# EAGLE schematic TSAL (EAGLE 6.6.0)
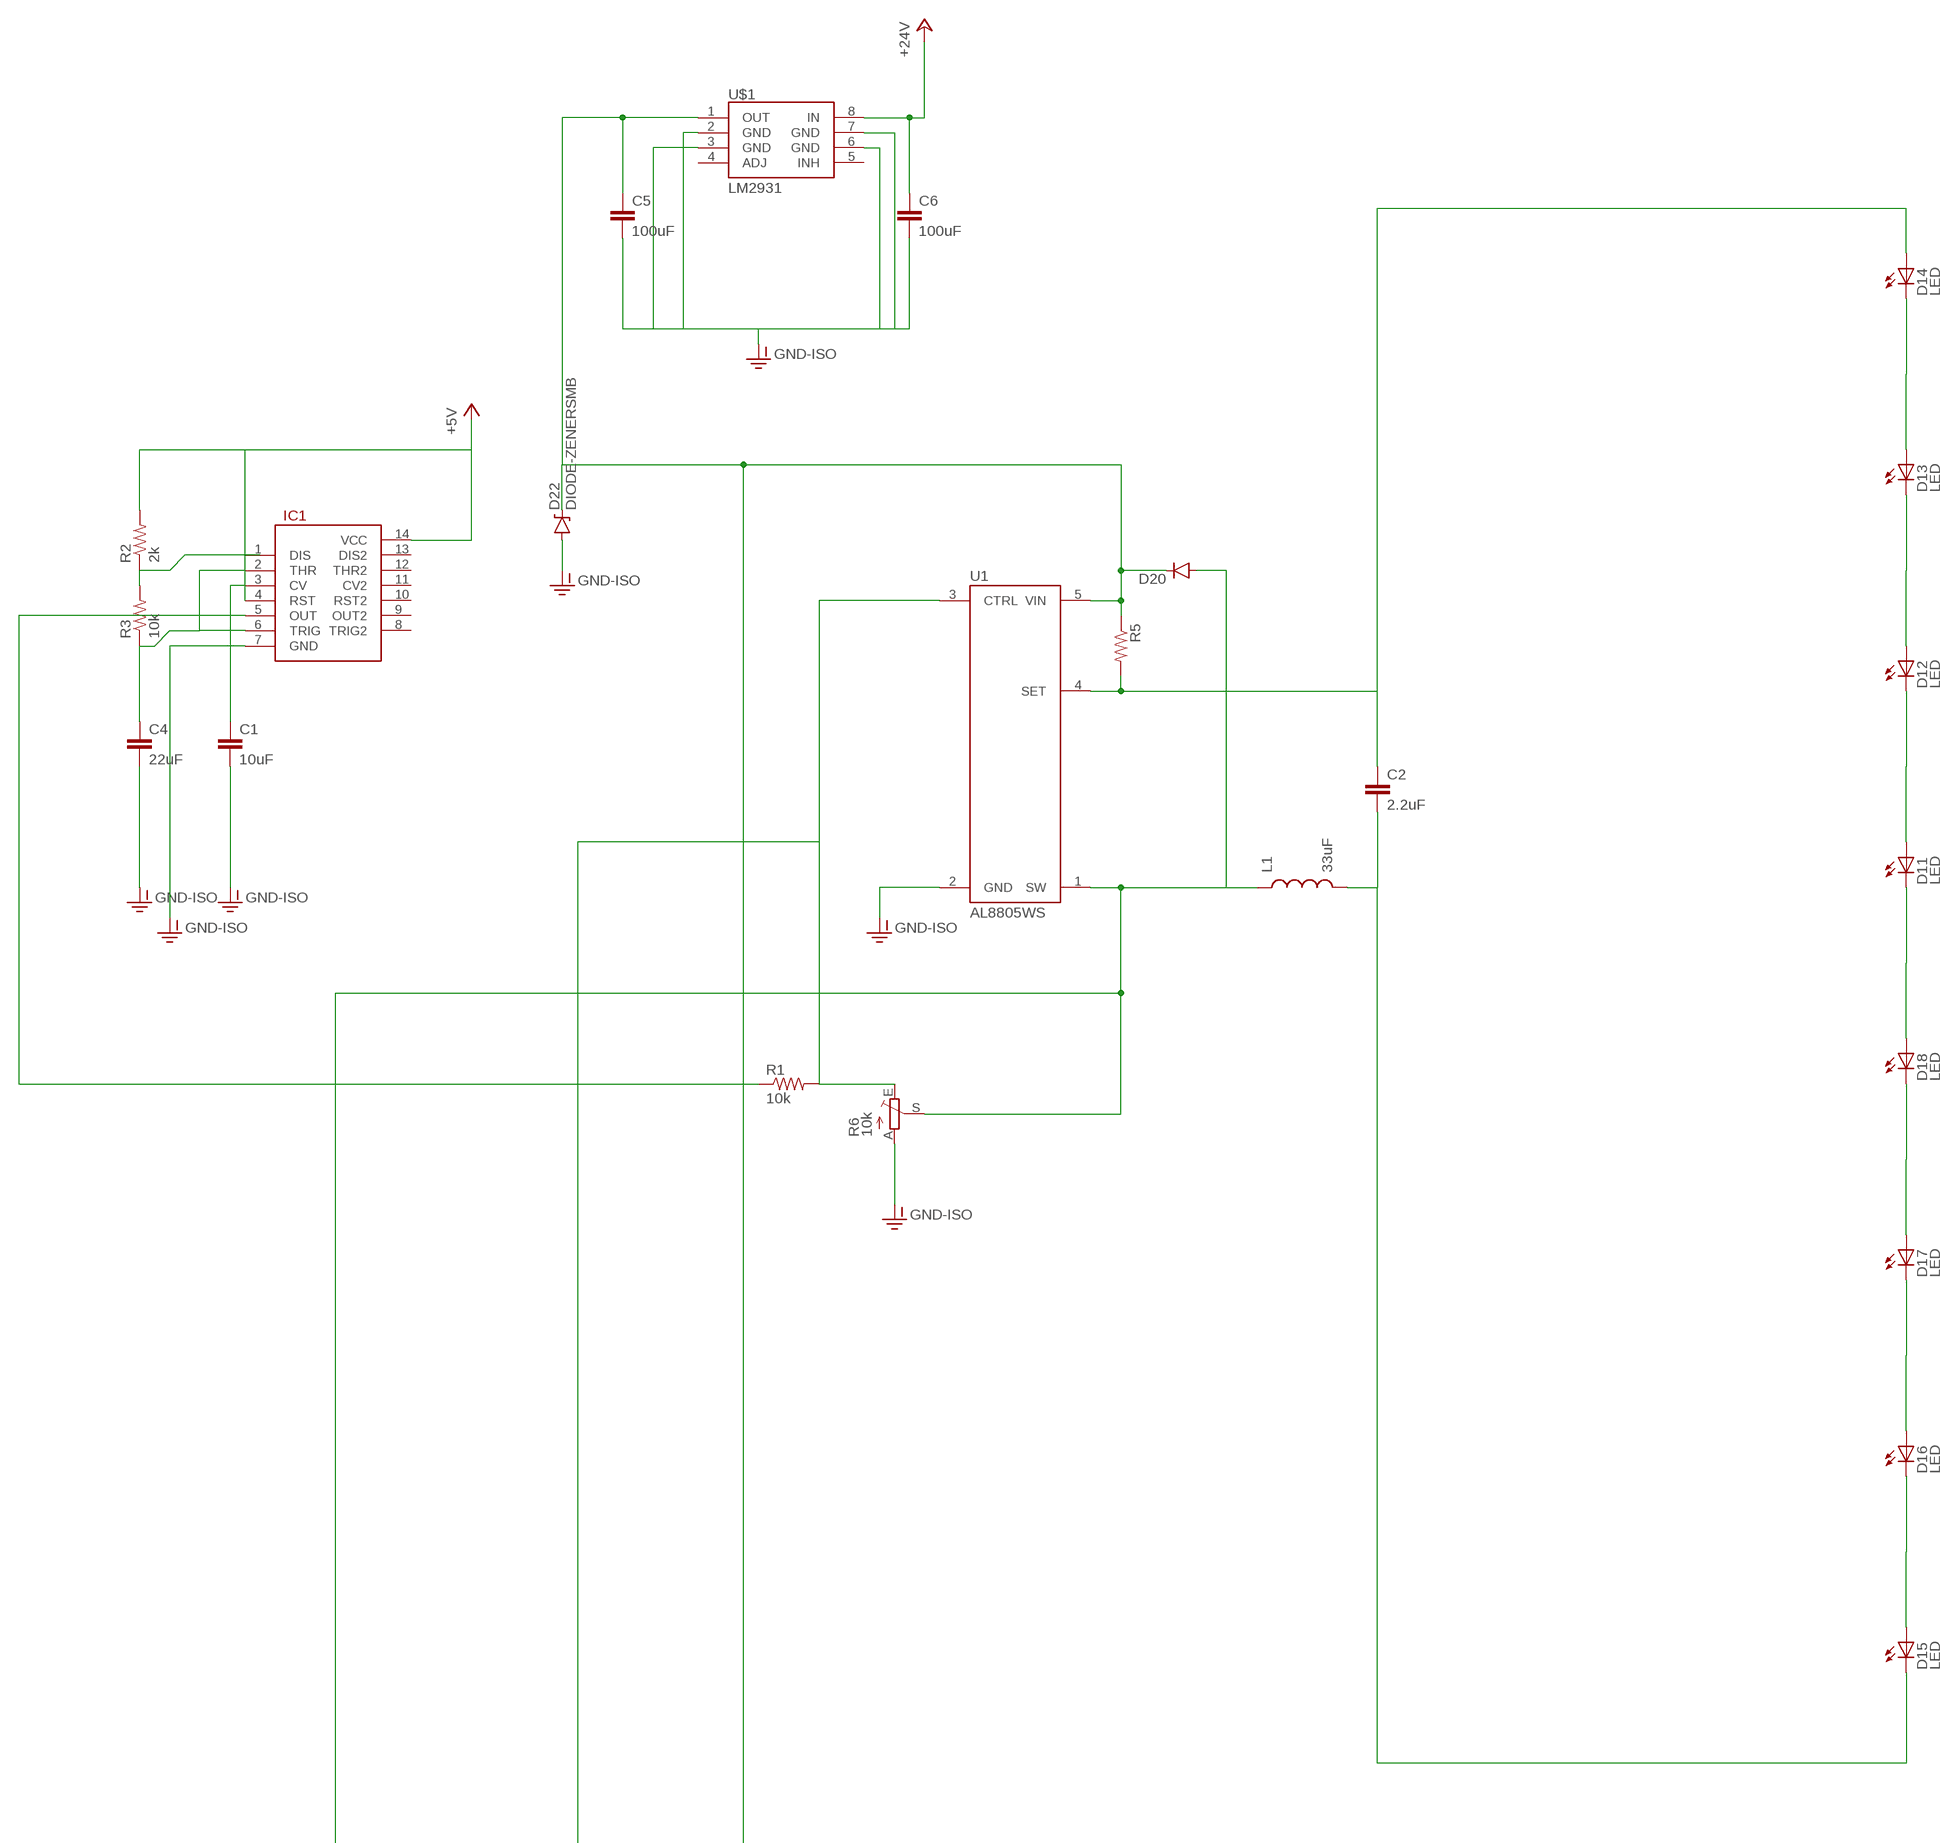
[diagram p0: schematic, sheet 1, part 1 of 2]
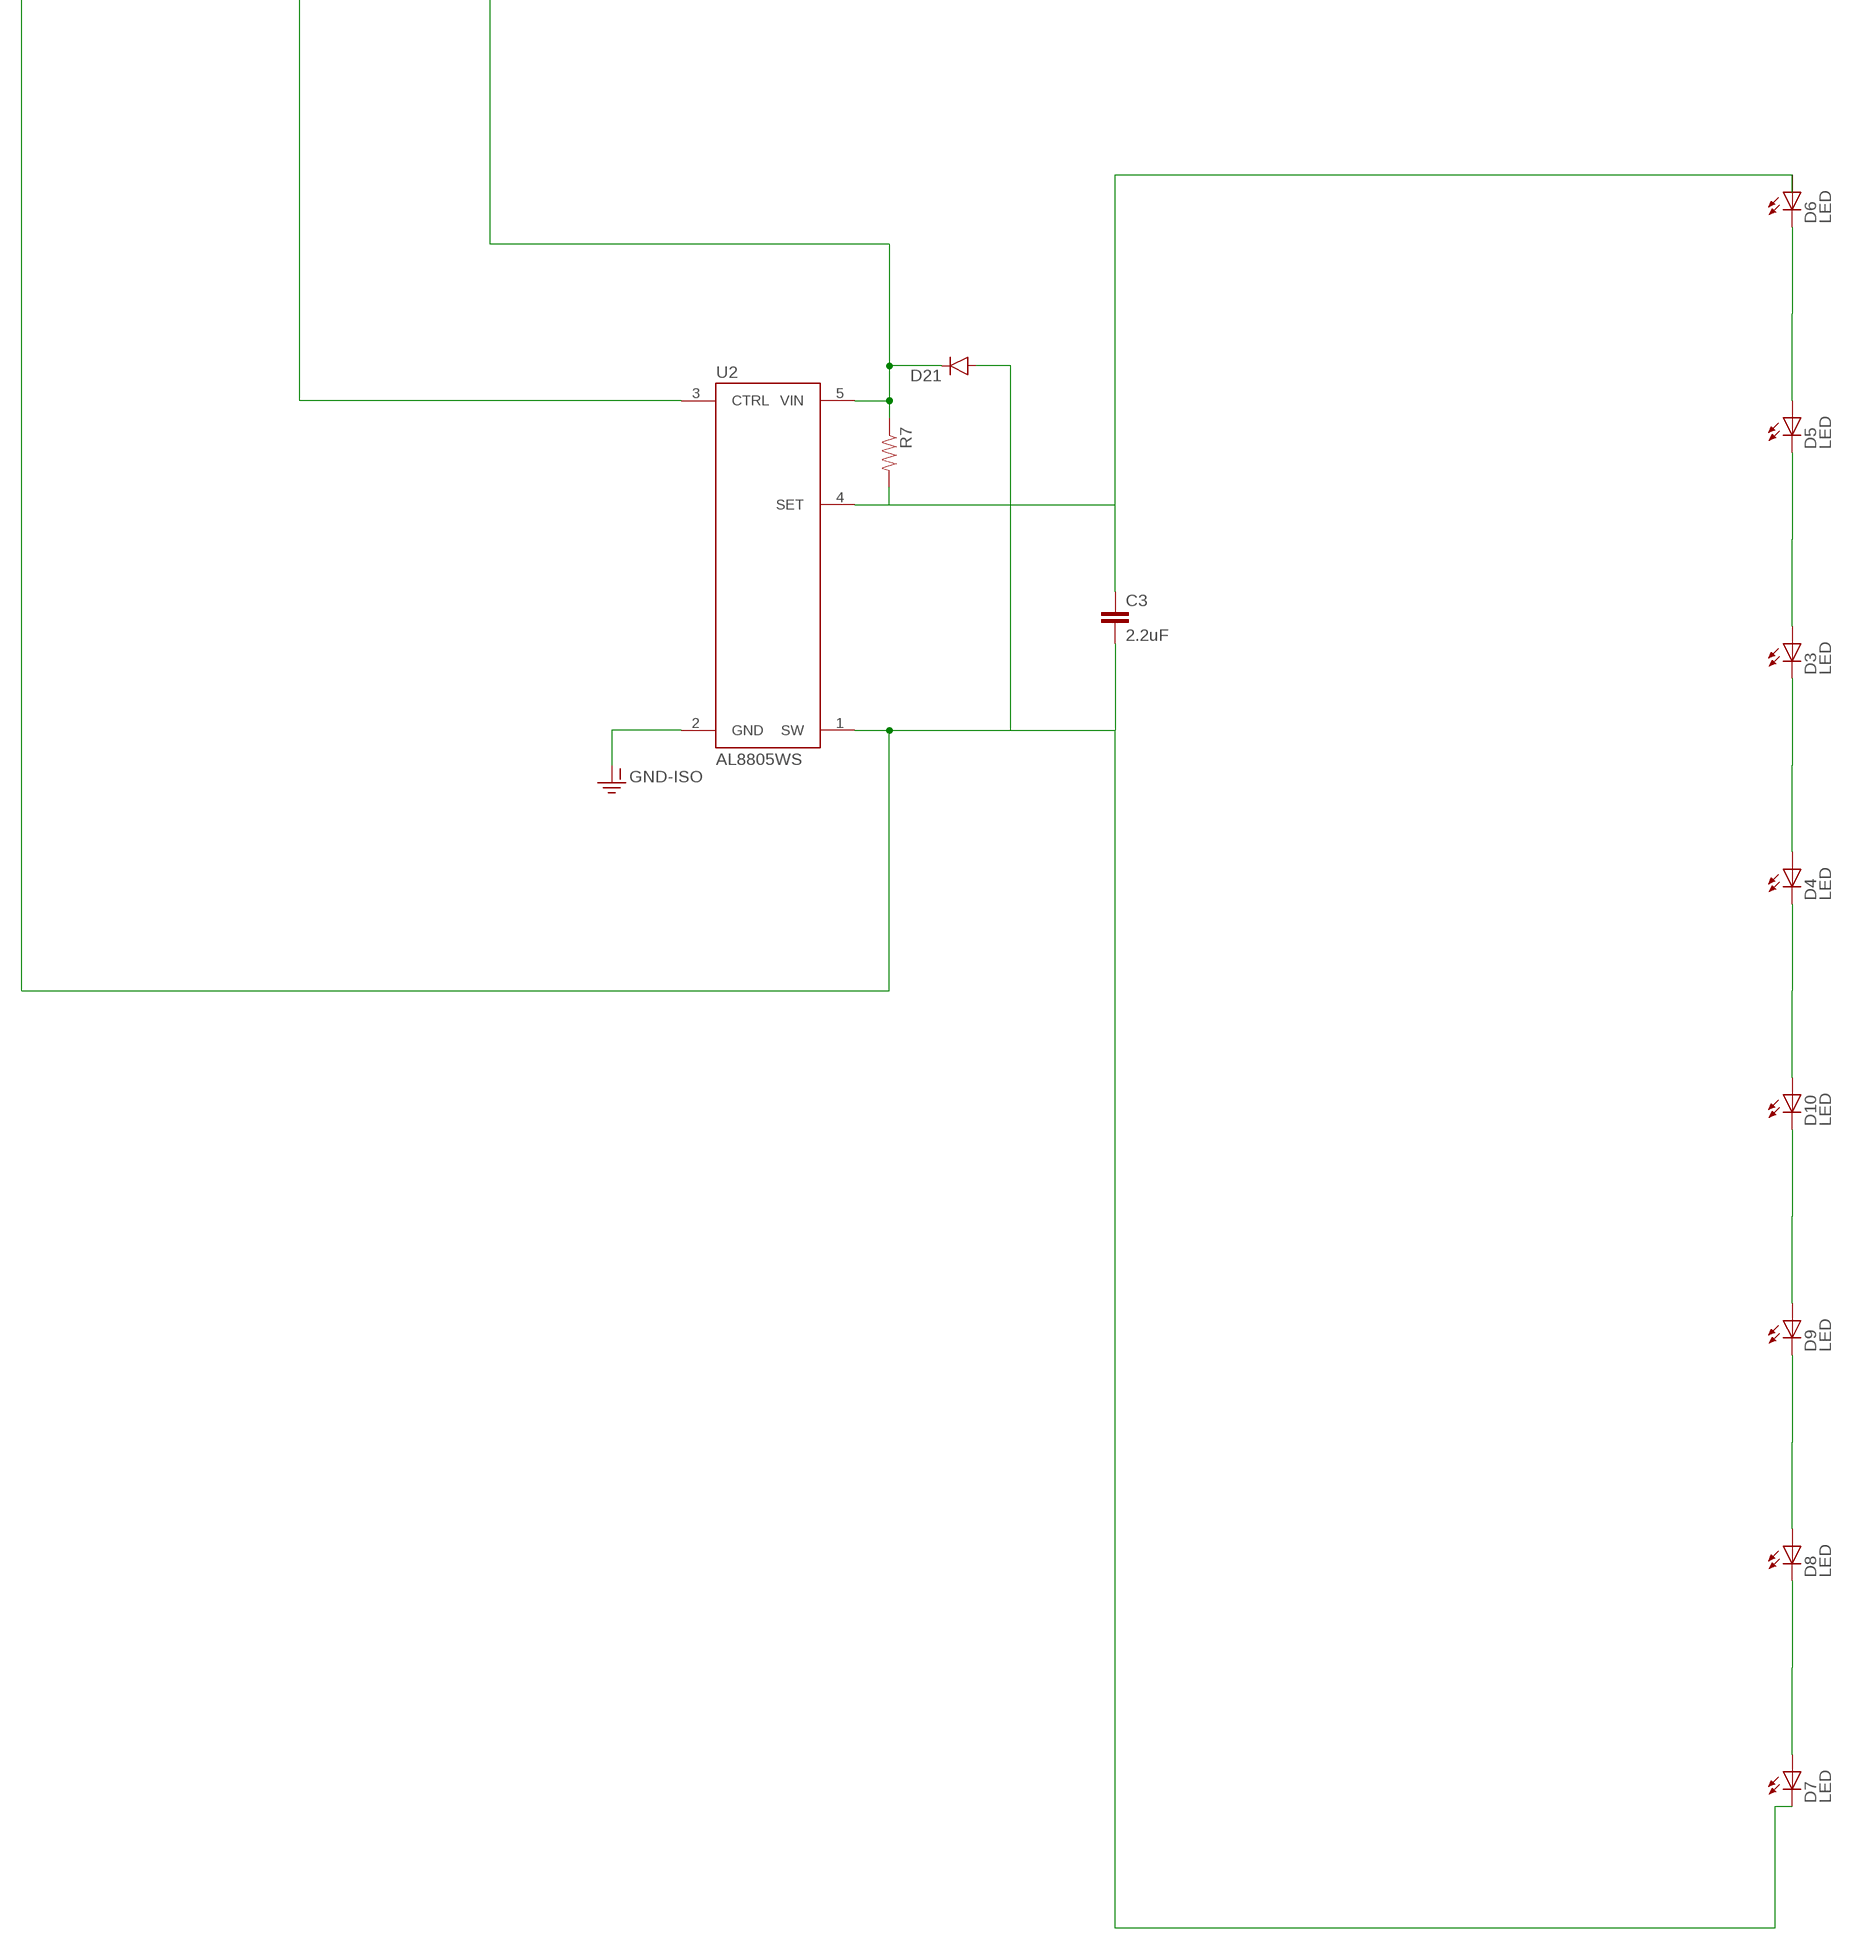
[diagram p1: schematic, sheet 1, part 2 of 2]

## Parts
C1  10uF  CAP0805  [0805]
C2  2.2uF  CAP0805  [0805]
C3  2.2uF  CAP0805  [0805]
C4  22uF  CAP0805  [0805]
C5  100uF  CAP0805  [0805]
C6  100uF  CAP0805  [0805]
D3  LED  [LED-SM]
D4  LED  [LED-SM]
D5  LED  [LED-SM]
D6  LED  [LED-SM]
D7  LED  [LED-SM]
D8  LED  [LED-SM]
D9  LED  [LED-SM]
D10  LED  [LED-SM]
D11  LED  [LED-SM]
D12  LED  [LED-SM]
D13  LED  [LED-SM]
D14  LED  [LED-SM]
D15  LED  [LED-SM]
D16  LED  [LED-SM]
D17  LED  [LED-SM]
D18  LED  [LED-SM]
D20  DIODESMB  [SMB-DIODE]
D21  DIODESMB  [SMB-DIODE]
D22  DIODE-ZENERSMB  [SMB-DIODE]
IC1  556  [DIL14]
L1  33uF  INDUCTOR0805  [0805]
R1  10k  RESISTOR0805-RES  [0805]
R2  2k  RESISTOR0805-RES  [0805]
R3  10k  RESISTOR0805-RES  [0805]
R5  RESISTOR0805-RES  [0805]
R6  10k  TRIM_EU-B25P  [B25P]
R7  RESISTOR0805-RES  [0805]
U1  AL8805WS  AL8805  [SOT23-5]
U2  AL8805WS  AL8805  [SOT23-5]
U$1  LM2931  [SO08]

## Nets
+5V: IC1.4(RST) IC1.14(VCC) R2.2
+24V: C6.1 U$1.8(IN)
GND-ISO: C1.2 C4.2 C5.2 C6.2 D22.A IC1.7(GND) R6.A U1.2(GND) U2.2(GND) U$1.2(GND) U$1.3(GND) U$1.6(GND) U$1.7(GND)
N$1: C3.1 D6.A R7.2 U2.4(SET)
N$2: IC1.5(OUT) R1.1
N$3: D4.A
N$4: C1.1 IC1.3(CV)
N$5: R2.1 R3.2
N$6: D4.C
N$7: C3.2 D7.C D20.A D21.A L1.1 R6.S U1.1(SW) U2.1(SW)
N$8: C2.1 D14.A R5.2 U1.4(SET)
N$10: C4.1 IC1.2(THR) IC1.6(TRIG) R3.1
N$11: D3.A
N$12: D3.C
N$13: D5.A
N$14: R1.2 R6.E U1.3(CTRL) U2.3(CTRL)
N$15: D5.C
N$17: D6.C
N$18: D7.A
N$19: C2.2 D15.C L1.2
N$20: D8.A
N$21: D8.C
N$22: D9.A
N$23: D9.C
N$24: D10.A
N$25: D10.C
N$26: D11.A
N$27: D11.C
N$28: D12.A
N$29: D12.C
N$30: D13.A
N$31: D13.C
N$33: D14.C
N$34: D15.A
N$35: C5.1 D20.C D21.C D22.C R5.1 R7.1 U1.5(VIN) U2.5(VIN) U$1.1(OUT)
N$36: D16.A
N$37: D16.C
N$38: D17.A
N$39: D17.C
N$40: D18.A
N$41: D18.C
Unconnected: IC1.1(DIS) IC1.8(TRIG2) IC1.9(OUT2) IC1.10(RST2) IC1.11(CV2) IC1.12(THR2) IC1.13(DIS2) U$1.4(ADJ) U$1.5(INH)

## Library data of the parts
C1-C6 = SparkFun-Capacitors:CAP: Capacitor
D3-D18 = FSAE Eletric:LED
D20 D21 = SparkFun-DiscreteSemi:DIODE: Diode; PROD_ID: DIO-09646
D22 = SparkFun-DiscreteSemi:DIODE-ZENER: Zener Diode
IC1 = SparkFun-AnalogIC:556: Dual timer circuit (2 555 timers in one package)
L1 = SparkFun-Passives:INDUCTOR: Inductors
R1-R3 R5 R7 = SparkFun-Passives:RESISTOR: Resistor
R6 = pot:TRIM_EU-: POTENTIOMETER
U1 U2 = SparkFun-PowerIC:AL8805: Constant current LED driver PWM-able 1MHz switch freq 6V-36V Up to 1A LED current; PROD_ID: IC-11626
U$1 = SparkFun-PowerIC:LM2931: LDO regulator with reverse battery protection- very durable!

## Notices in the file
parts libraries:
SparkFun-PowerIC: Licensing: Creative Commons ShareAlike 4.0 International - https://creativecommons.org/licenses/by-sa/4.0
